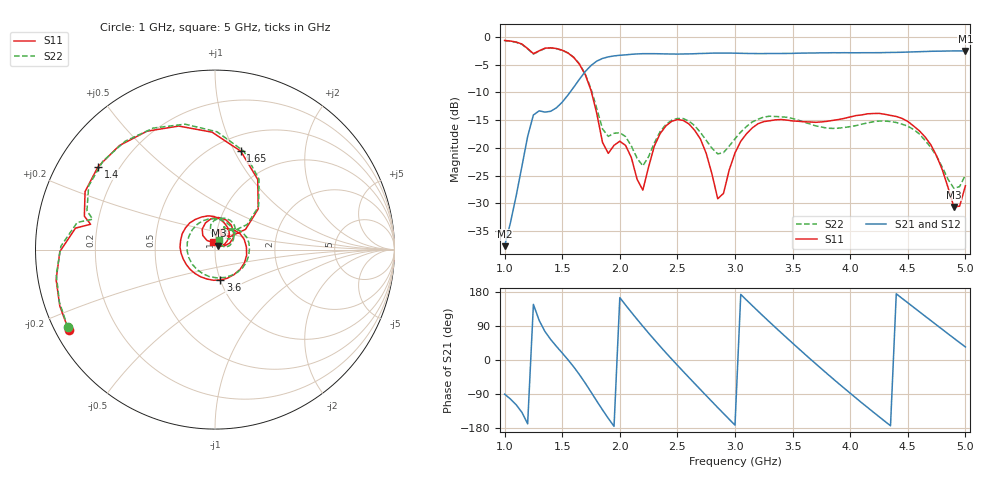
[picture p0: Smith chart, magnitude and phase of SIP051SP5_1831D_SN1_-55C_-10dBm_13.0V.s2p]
# GHz  S  dB  R  50
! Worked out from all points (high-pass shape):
!   81 points, 1 GHz to 5 GHz, reference 50 ohm
!   highest |S21| = -2.51 dB at 5 GHz (marker M1); lowest = -37.7 dB at 1 GHz (marker M2)
!   |S21| within 3 dB of the highest: 1.733 GHz to end of sweep
!   lowest |S11| = -30.7 dB at 4.9 GHz (marker M3), VSWR 1.06, Z = 51.9 + j2.28 ohm
!   |S11| at or under -10 dB: 1.755 GHz to end of sweep
!   |S22| runs from -27.3 to -0.7 dB; largest |S21 - S12| = 0.0019
!   S11 on the Smith chart (normalised r, x): 1 GHz: 0.04, -0.26; 1.4 GHz: 0.12, +0.31; 1.65 GHz: 0.66, +1.06; 3.6 GHz: 1.00, -0.35; 5 GHz: 0.97, +0.09
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1  -0.62 -151.2  -37.74 -90.2  -37.76 -91.4  -0.66 -152.1
1.25  -3.01 168.5  -14.07 146.9  -14.06 146.8  -3.07 166.0
1.4  -1.95 144.6  -13.40 54.1  -13.39 54.1  -1.99 141.8
1.55  -2.88 106.4  -10.47 0.7  -10.47 0.6  -2.87 103.4
1.65  -4.93 75.3  -7.60 -38.8  -7.60 -38.8  -4.86 73.6
1.7  -6.79 58.7  -6.24 -60.9  -6.25 -61.0  -6.69 58.0
1.85  -19.02 40.3  -3.87 -131.7  -3.87 -131.7  -16.58 44.8
2  -18.80 76.2  -3.30 164.6  -3.29 164.6  -17.27 66.1
2.2  -27.63 105.5  -3.01 89.1  -3.02 89.1  -23.25 81.6
2.35  -17.43 122.1  -3.02 36.1  -3.02 36.2  -17.08 99.8
2.5  -14.90 83.8  -3.08 -13.9  -3.07 -13.8  -14.70 71.4
2.7  -18.41 32.2  -2.97 -78.1  -2.97 -78.1  -17.21 37.5
2.85  -29.18 40.1  -2.90 -125.5  -2.91 -125.5  -21.09 44.2
3  -20.91 82.7  -2.92 -171.8  -2.91 -171.8  -18.36 58.3
3.3  -15.11 4.8  -2.98 100.2  -2.99 100.2  -14.29 11.1
3.6  -15.29 -79.9  -2.90 17.2  -2.91 17.1  -15.37 -57.5
3.7  -15.39 -105.6  -2.88 -9.7  -2.88 -9.7  -16.03 -85.7
4  -14.42 -174.0  -2.84 -87.7  -2.84 -87.7  -16.17 -178.0
4.35  -14.14 112.3  -2.78 -173.5  -2.80 -173.5  -15.24 89.4
4.65  -18.02 50.9  -2.62 115.8  -2.62 115.7  -18.66 28.7
4.9  -30.66 48.6  -2.51 57.5  -2.51 57.4  -27.29 33.5
5  -26.86 105.9  -2.51 34.4  -2.51 34.3  -24.92 64.4
